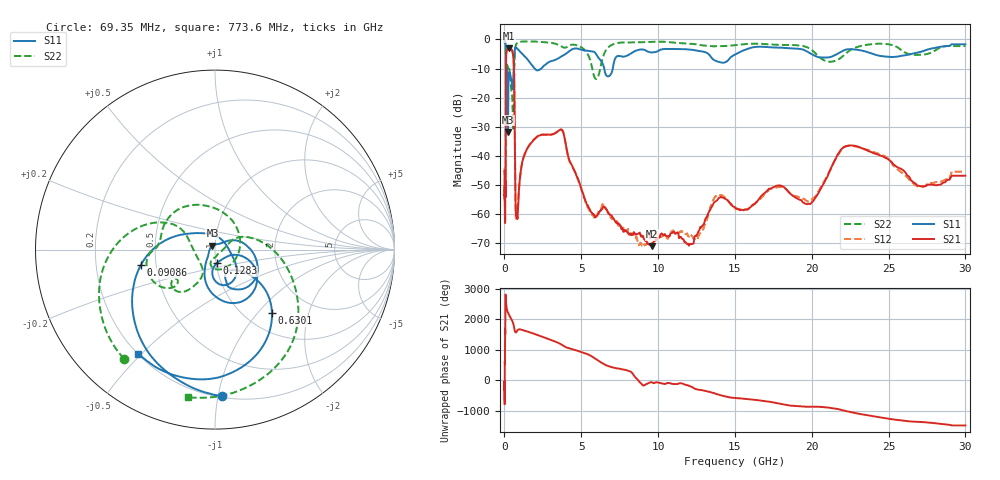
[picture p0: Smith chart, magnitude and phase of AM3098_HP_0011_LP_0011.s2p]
! Date/Time: Thu, Feb 28, 2019 8:33 AM
! Network Analyzer: Agilent Technologies E8364B Rev: A.07.50.67
! Sweep from 0.010 to 30.000 GHz, 1601 Points, Sweep Type: LOG
! Power Supply: 5.022 V, 0.002 A
# Hz S DB R 50
!freq MagS11 AngS11 MagS21 AngS21 MagS12 AngS12 MagS22 AngS22
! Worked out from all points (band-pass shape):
!   1601 points, 10 MHz to 30 GHz, reference 50 ohm
!   highest |S21| = -3.05 dB at 266.5 MHz (marker M1); lowest = -71.0 dB at 9.586 GHz (marker M2)
!   |S21| within 3 dB of the highest: 107.7 MHz to 576.7 MHz (469 MHz wide, 137 % of centre)
!   lowest |S11| = -31.8 dB at 228.2 MHz (marker M3), VSWR 1.05, Z = 48.5 + j2.07 ohm
!   |S11| at or under -10 dB: 175.5 MHz to 598.3 MHz (422.9 MHz wide, 109 % of centre); 1.976 GHz to 2.398 GHz (422.1 MHz wide, 19.3 % of centre); 6.495 GHz to 7.05 GHz (555.8 MHz wide, 8.21 % of centre)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
!   |S22| runs from -30.6 to -0.5 dB; largest |S21 - S12| = 0.01
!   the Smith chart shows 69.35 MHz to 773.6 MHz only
!   S11 on the Smith chart (normalised r, x): 69.35 MHz: 0.21, -1.03; 90.86 MHz: 0.41, -0.09; 128.3 MHz: 1.01, -0.16; 630.1 MHz: 1.31, -1.20; 773.6 MHz: 0.20, -0.49
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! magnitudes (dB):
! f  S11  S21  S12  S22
! 10 MHz  -0.3  -45.1  -44.1  -0.5
! 38.04 MHz  -0.5  -58.5  -59.9  -0.9
! 69.35 MHz  -1.7  -54.2  -52.4  -2.0
! 90.86 MHz  -7.5  -20.9  -20.7  -8.6
! 100.9 MHz  -23.5  -8.1  -8.1  -17.1
! 128.3 MHz  -22.2  -4.2  -4.2  -11.0
! 144.7 MHz  -14.2  -3.7  -3.6  -10.4
! 186.8 MHz  -11.5  -3.5  -3.5  -8.2
! 228.2 MHz  -31.8  -3.1  -3.1  -9.8
! 266.5 MHz  -14.9  -3.0  -3.0  -10.2
! 550.5 MHz  -15.9  -5.0  -4.9  -27.2
! 630.1 MHz  -6.4  -12.8  -12.7  -13.1
! 717.7 MHz  -2.7  -55.0  -55.7  -2.4
! 773.6 MHz  -2.8  -60.1  -61.3  -1.6
! 2.084 GHz  -10.5  -33.6  -33.6  -0.7
! 3.723 GHz  -5.8  -31.0  -30.9  -2.4
! 5.959 GHz  -5.0  -60.8  -60.9  -13.6
! 7.926 GHz  -5.7  -65.8  -65.8  -1.0
! 9.586 GHz  -4.5  -71.0  -66.7  -0.8
! 19.7 GHz  -4.2  -56.6  -55.5  -2.7
! 22.56 GHz  -3.3  -36.4  -36.5  -3.5
! 30 GHz  -1.7  -46.8  -45.4  -2.3
